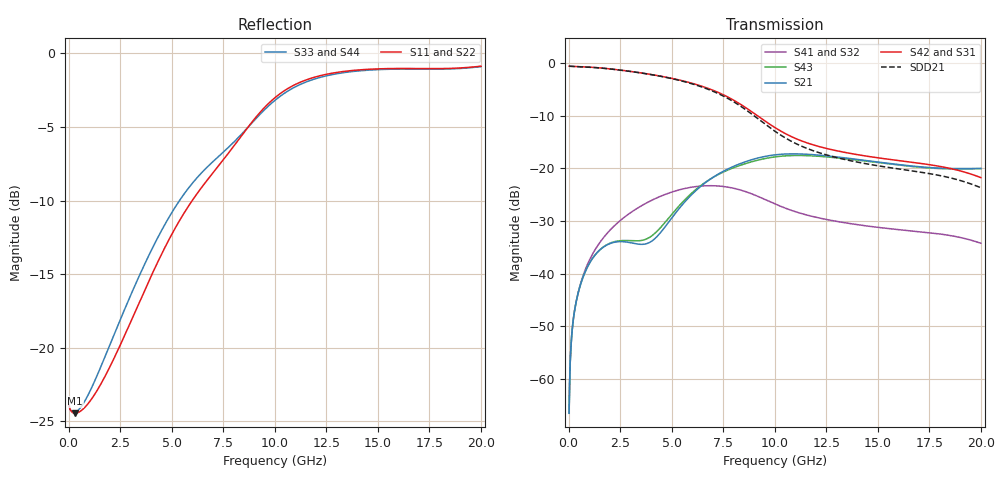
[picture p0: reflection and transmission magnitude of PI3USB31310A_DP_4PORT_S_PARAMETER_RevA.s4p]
! NPort=4 DATA=800 NOISE=0 GROUPDELAY=0 COMPLEX_DATAFORMAT=POLAR
! NumOfBlock=1 NumOfParam=0
! .MODEL Smodel S TSTONEFILE=PI3USB31310A_DP_4PORT_S_PARAMETER_RevA.s4p TYPE=S
!  -- The above .MODEL line can be used for the S element in the netlist.
!  Port definition:
!  Port1 = INPUT+
!  Port2 = INPUT-
!  Port3 = OUTPUT+
!  Port4 = OUTPUT-
# Hz S MA R  50
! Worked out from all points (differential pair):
!   800 points, 25 MHz to 20 GHz, reference 50 ohm
!   strongest paths, dB at 25 MHz, 5.025 GHz, 10.03 GHz, 15.03 GHz, 20 GHz:
!     S42: -0.6, -2.9, -12.3, -18.0, -21.8
!     S31: -0.6, -2.9, -12.3, -18.0, -21.8
!     S21: -66.5, -29.3, -17.4, -18.8, -20.0
!     S43: -66.5, -28.7, -17.8, -18.9, -20.1
!     S41: -66.5, -24.5, -26.8, -31.2, -34.2
!     S32: -66.5, -24.5, -26.8, -31.2, -34.2
!   taken as a pair (ports 2,1 in; 4,3 out), SDD21 dB: -0.6, -3.0, -13.0, -19.5, -23.7
!   lowest |S11| = -24.5 dB at 325 MHz (marker M1), VSWR 1.13, Z = 56.4 - j0.222 ohm
!   |S11| at or under -10 dB: start of sweep to 5.995 GHz
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2.5e7  0.06366 -2.0  0.0004739 87.3  0.9322 -0.7  0.000471 87.2
       0.0004739 87.3  0.06366 -2.0  0.000471 87.2  0.9322 -0.7
       0.9322 -0.7  0.0004711 87.2  0.06367 -1.8  0.0004739 87.3
       0.0004711 87.2  0.9322 -0.7  0.0004739 87.3  0.06367 -1.8
3.25e8  0.0599 -1.9  0.004885 73.4  0.9265 -7.3  0.004893 72.7
        0.004885 73.4  0.0599 -1.9  0.004893 72.7  0.9265 -7.3
        0.9265 -7.3  0.004893 72.7  0.06042 1.4  0.004884 73.6
        0.004893 72.7  0.9265 -7.3  0.004884 73.6  0.06042 1.4
1.45e9  0.07293 -2.5  0.0163 59.9  0.8998 -31.9  0.01892 54.7
        0.0163 59.9  0.07293 -2.5  0.01892 54.7  0.8998 -31.9
        0.8999 -31.9  0.01892 54.8  0.08259 6.3  0.01635 61.0
        0.01892 54.8  0.8999 -31.9  0.01635 61.0  0.08259 6.3
3.425e9  0.1424 -12.2  0.019 57.3  0.8092 -73.6  0.04279 13.6
         0.019 57.3  0.1424 -12.2  0.04279 13.6  0.8092 -73.6
         0.8094 -73.6  0.0428 13.6  0.1754 -9.2  0.0205 60.1
         0.0428 13.6  0.8094 -73.6  0.0205 60.1  0.1754 -9.2
6.8e9  0.3771 -42.4  0.07705 78.3  0.5702 -146.2  0.06829 -69.0
       0.07705 78.3  0.3771 -42.4  0.06829 -69.0  0.5702 -146.2
       0.5703 -146.1  0.06831 -69.0  0.416 -47.8  0.07735 73.6
       0.06831 -69.0  0.5703 -146.1  0.07735 73.6  0.416 -47.8
1.1975e10  0.8321 -90.5  0.1341 9.6  0.1643 147.2  0.03433 -163.7
           0.1341 9.6  0.8321 -90.5  0.03433 -163.7  0.1643 147.2
           0.1644 147.3  0.03435 -163.6  0.8205 -91.4  0.1306 9.7
           0.03435 -163.6  0.1644 147.3  0.1306 9.7  0.8205 -91.4
2e10  0.9052 -125.7  0.09972 -25.0  0.08143 54.3  0.01938 83.8
      0.09972 -25.0  0.9052 -125.7  0.01938 83.8  0.08143 54.3
      0.08152 54.4  0.0194 83.9  0.9018 -125.8  0.09915 -24.7
      0.0194 83.9  0.08152 54.4  0.09915 -24.7  0.9018 -125.8
